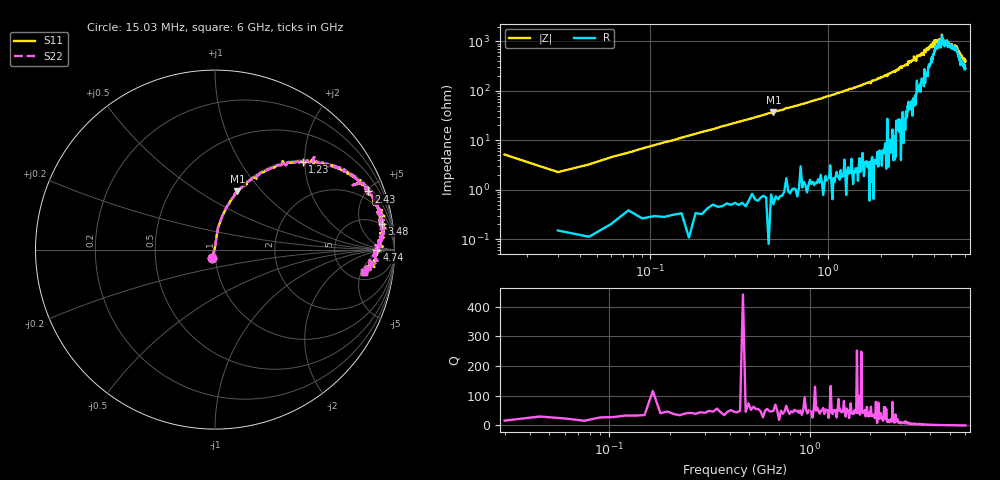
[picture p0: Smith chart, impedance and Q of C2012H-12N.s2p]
!	Network	Analyzer	HP8753E.07.74:	Oct	30	2002	Serial	No.	JP38451487
!	Hewlett-Packard
!	28	Aug	2009	9:42:43
!	Frequency	S11	S21	S12	S22
#	HZ	S	RI	R	50
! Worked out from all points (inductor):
!   400 points, 15.03 MHz to 6 GHz, reference 50 ohm
!   read as one part in series: L = 11.9 nH near 45.03 MHz
!   highest Q = 54.2 at 495 MHz (marker M1), where L = 12 nH
!   self-resonance near 4.597 GHz
!   S11 on the Smith chart (normalised r, x): 15.03 MHz: 0.96, -0.10; 1.23 GHz: 1.04, +1.96; 2.43 GHz: 1.30, +5.14; 3.48 GHz: 4, +11; 4.74 GHz: 19, -0; 6 GHz: 6.68, -5.60
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1.502992e7  -0.0159 -0.0492  1.02 0.0492  1.02 0.0492  -0.0159 -0.0492
3.002985e7  0.00201 0.0226  0.998 -0.0226  0.998 -0.0226  0.00201 0.0226
9.002955e7  0.00742 0.0675  0.993 -0.0675  0.993 -0.0675  0.00742 0.0675
1.650292e8  0.0164 0.122  0.984 -0.122  0.984 -0.122  0.0164 0.122
4.950275e8  0.125 0.324  0.875 -0.324  0.875 -0.324  0.125 0.324
1.020025e9  0.386 0.476  0.614 -0.476  0.614 -0.476  0.386 0.476
1.230024e9  0.489 0.49  0.511 -0.49  0.511 -0.49  0.489 0.49
2.01002e9  0.771 0.405  0.229 -0.405  0.229 -0.405  0.771 0.405
2.430018e9  0.855 0.324  0.145 -0.324  0.145 -0.324  0.855 0.324
3.015015e9  0.931 0.219  0.0693 -0.219  0.0693 -0.219  0.931 0.219
3.480013e9  0.93 0.145  0.0704 -0.145  0.0704 -0.145  0.93 0.145
3.91501e9  0.92 0.0925  0.0799 -0.0925  0.0799 -0.0925  0.92 0.0925
4.00501e9  0.94 0.066  0.0599 -0.066  0.0599 -0.066  0.94 0.066
4.365008e9  0.911 0.0502  0.0889 -0.0502  0.0889 -0.0502  0.911 0.0502
4.425008e9  0.935 0.0173  0.0654 -0.0173  0.0654 -0.0173  0.935 0.0173
4.455008e9  0.905 0.0266  0.0948 -0.0266  0.0948 -0.0266  0.905 0.0266
4.485008e9  0.92 0.0178  0.0801 -0.0178  0.0801 -0.0178  0.92 0.0178
4.740006e9  0.901 -0.0018  0.099 0.0018  0.099 0.0018  0.901 -0.0018
5.010005e9  0.894 -0.0214  0.106 0.0214  0.106 0.0214  0.894 -0.0214
5.385003e9  0.894 -0.0454  0.106 0.0454  0.106 0.0454  0.894 -0.0454
5.625002e9  0.865 -0.114  0.135 0.114  0.135 0.114  0.865 -0.114
6e9  0.83 -0.124  0.17 0.124  0.17 0.124  0.83 -0.124
